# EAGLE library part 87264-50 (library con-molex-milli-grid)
RECEPTACAL
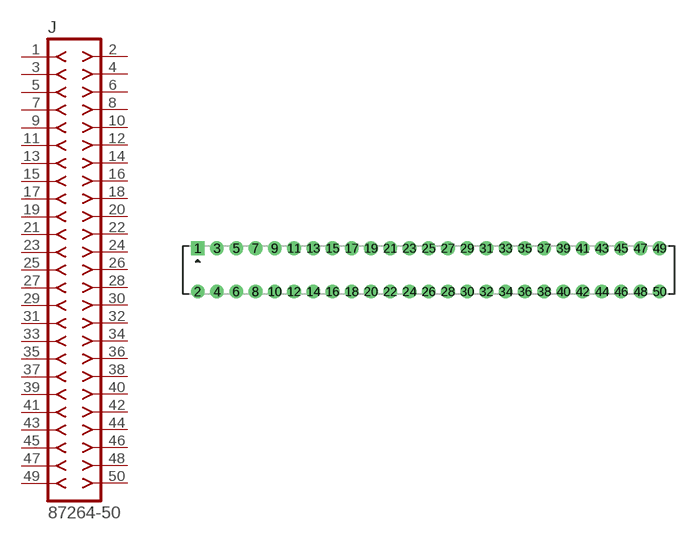
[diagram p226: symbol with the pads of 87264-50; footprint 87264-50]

Designator prefix J

## 87264-50  [87264-50]
1  1  pas
2  2  pas
3  3  pas
4  4  pas
5  5  pas
6  6  pas
7  7  pas
8  8  pas
9  9  pas
10  10  pas
11  11  pas
12  12  pas
13  13  pas
14  14  pas
15  15  pas
16  16  pas
17  17  pas
18  18  pas
19  19  pas
20  20  pas
21  21  pas
22  22  pas
23  23  pas
24  24  pas
25  25  pas
26  26  pas
27  27  pas
28  28  pas
29  29  pas
30  30  pas
31  31  pas
32  32  pas
33  33  pas
34  34  pas
35  35  pas
36  36  pas
37  37  pas
38  38  pas
39  39  pas
40  40  pas
41  41  pas
42  42  pas
43  43  pas
44  44  pas
45  45  pas
46  46  pas
47  47  pas
48  48  pas
49  49  pas
50  50  pas

## Footprint 87264-50 (pad centres in mm)
RECEPTACAL Dual Row, Side Entry
drill 0.914 square: 1 -24,2.25
drill 0.914: 2 -24,-2.25; 3 -22,2.25; 4 -22,-2.25; 5 -20,2.25; 6 -20,-2.25; 7 -18,2.25; 8 -18,-2.25; 9 -16,2.25; 10 -16,-2.25; 11 -14,2.25; 12 -14,-2.25; 13 -12,2.25; 14 -12,-2.25; 15 -10,2.25; 16 -10,-2.25; 17 -8,2.25; 18 -8,-2.25; 19 -6,2.25; 20 -6,-2.25; 21 -4,2.25; 22 -4,-2.25; 23 -2,2.25; 24 -2,-2.25; 25 0,2.25; 26 0,-2.25; 27 2,2.25; 28 2,-2.25; 29 4,2.25; 30 4,-2.25; 31 6,2.25; 32 6,-2.25; 33 8,2.25; 34 8,-2.25; 35 10,2.25; 36 10,-2.25; 37 12,2.25; 38 12,-2.25; 39 14,2.25; 40 14,-2.25; 41 16,2.25; 42 16,-2.25; 43 18,2.25; 44 18,-2.25; 45 20,2.25; 46 20,-2.25; 47 22,2.25; 48 22,-2.25; 49 24,2.25; 50 24,-2.25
